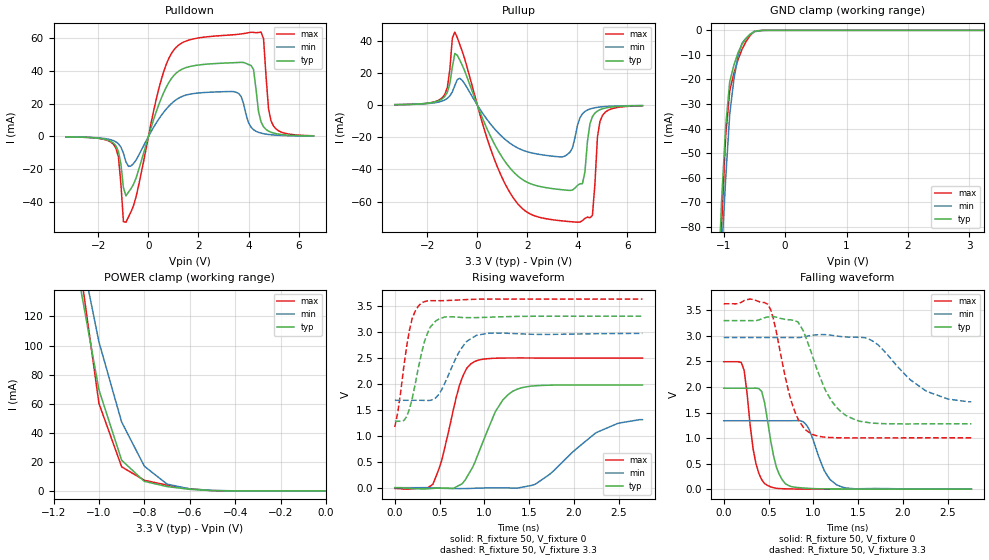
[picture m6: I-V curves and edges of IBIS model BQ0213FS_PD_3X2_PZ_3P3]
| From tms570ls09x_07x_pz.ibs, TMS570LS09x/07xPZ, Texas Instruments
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|   Model Cell BQ0213FS_PD_3X2_PZ_3P3
|BQ0213FS_PD_3X2_PZ_3P3
[Model]   BQ0213FS_PD_3X2_PZ_3P3
Model_type   I/O
Polarity   Non-Inverting
Enable   Active-Low
Vinl =  1.25
Vinh =  1.65
Cref =  15.0001pF
Rref =  101.0000M
Vref =  0V
Vmeas =  1.65
C_comp   1.2p   1.2p   1.2p
[Model Spec]
Vinl   1.25   1.12   1.38
Vinh   1.65   1.45   1.75
[Temperature Range]   25   155   -40
[Voltage Range]   3.3   2.97   3.63
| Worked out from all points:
|   slope of the pulldown table from 0 to 0.495 V, typ, clamps not added: 22 ohm
|   slope of the pullup table from 0 to 0.495 V, typ, clamps not added: 26.9 ohm
|   GND clamp passes 1 mA (typ) near -0.53 V on its own axis
|   POWER clamp passes 1 mA (typ) near -0.59 V on its own axis
|   rising waveform, R_fixture 50, V_fixture 0: 20-80 % time 297ps typ, 507ps min, 210ps max; typ from 0 V to 1.98 V
|   rising waveform, R_fixture 50, V_fixture 3.3: 20-80 % time 159ps typ, 218ps min, 127ps max; typ from 1.28 V to 3.3 V
|   falling waveform, R_fixture 50, V_fixture 0: 20-80 % time 129ps typ, 181ps min, 108ps max; typ from 1.98 V to 0.001 V
|   falling waveform, R_fixture 50, V_fixture 3.3: 20-80 % time 290ps typ, 442ps min, 208ps max; typ from 3.3 V to 1.28 V
[POWER_clamp]
|   voltage   I(typ)   I(min)   I(max)
-3.3V     2.375A     2.63A      3.153A
-1.1V     156mA      180.2mA    173.4mA
-1.067V   127.2mA    154.3mA    135.6mA
-1.033V   98.41mA    128.4mA    97.92mA
-1V       69.61mA    102.5mA    60.2mA
-900mV    21.13mA    47.41mA    16.61mA
-800mV    6.576mA    17mA       7.309mA
-700mV    2.999mA    4.688mA    3.99mA
-600mV    1.087mA    1.404mA    1.425mA
-500mV    187uA      358.1uA    203.4uA
0V        311.4pA    5.945nA    272.3pA
[Pulldown]
|   voltage   I(typ)   I(min)   I(max)
-3.3V     -269.8uA   -248.1uA   -260.2uA
-1.4V     -4.056mA   -2.548mA   -4.78mA
-1.2V     -9.104mA   -4.482mA   -12.53mA
-900mV    -36.12mA   -15.43mA   -52.08mA
1V        36.78mA    21.07mA    52.28mA
3.5V      44.86mA    26.92mA    61.93mA
4.1V      43.14mA    5.644mA    63.29mA
4.5V      8.805mA    2.025mA    63.4mA
4.6V      5.861mA    1.678mA    59.29mA
4.8V      3.241mA    1.203mA    16.69mA
5V        2.072mA    900.6uA    6.272mA
6.6V      302.2uA    232.4uA    414.2uA
[Pullup]
|   voltage   I(typ)   I(min)   I(max)
-3.3V     296.7uA    284.3uA    270.4uA
-1.4V     3.996mA    2.582mA    4.655mA
-1.2V     8.017mA    4.201mA    10.97mA
-900mV    32.15mA    12.24mA    45.44mA
1.4V      -40.82mA   -24.72mA   -56.86mA
3.4V      -52.65mA   -32.22mA   -72.03mA
4V        -49.98mA   -12.64mA   -72.82mA
4.2V      -48.91mA   -5.386mA   -71.83mA
4.6V      -7.16mA    -1.965mA   -68.52mA
4.8V      -3.684mA   -1.373mA   -19.8mA
5V        -2.282mA   -1.01mA    -6.487mA
6.6V      -316.6uA   -254.8uA   -401.1uA
[GND_clamp]
|   voltage   I(typ)   I(min)   I(max)
-3.3V     -1.947A    -1.623A    -3.254A
-1.1V     -112mA     -127mA     -135.8mA
-1.033V   -69.61mA   -91.63mA   -80.19mA
-966.7mV  -39.23mA   -60.62mA   -43.11mA
-900mV    -20.86mA   -34.02mA   -24.52mA
-833.3mV  -14.26mA   -20.12mA   -17.61mA
-766.7mV  -9.194mA   -10.52mA   -12.01mA
-700mV    -5.668mA   -5.208mA   -7.706mA
-566.7mV  -1.566mA   -1.573mA   -2.055mA
-500mV    -402.3uA   -585.8uA   -459.7uA
-300mV    -821.9nA   -7.17uA    -404.6nA
3.233V    296.5pA    4.008uA    206.9pA
[Ramp]
| variable   typ   min   max
dV/dt_f   1.26115/0.2950033n  0.8126168/0.4782827n   1.631567/0.2134149n
dV/dt_r   1.201273/0.3013661n  0.8158071/0.535569n   1.515362/0.2079949n
R_load = 50
[Rising Waveform]
R_fixture = 50
V_fixture = 0
V_fixture_min = 0
V_fixture_max = 0
|   time   V(typ)   V(min)   V(max)
0s        -29.41uV   10.5uV     -14.61mV
424ps     -14.21mV   -3.24mV    63.63mV
524ps     -7.849mV   -11.94mV   525.3mV
720ps     47.03mV    -17.96mV   1.958V
888ps     465mV      -11.29mV   2.425V
1.124ns   1.469V     -3.041mV   2.491V
1.312ns   1.852V     -6.722mV   2.496V
1.568ns   1.961V     66.56mV    2.496V
2.24ns    1.977V     1.051V     2.495V
2.764ns   1.977V     1.309V     2.495V
[Rising Waveform]
R_fixture = 50
V_fixture = 3.3
V_fixture_min = 2.97
V_fixture_max = 3.63
|   time   V(typ)   V(min)   V(max)
0s        1.281V     1.682V     1.167V
100ps     1.291V     1.682V     2.323V
164ps     1.514V     1.682V     3.034V
228ps     1.997V     1.682V     3.398V
296ps     2.569V     1.681V     3.557V
392ps     3.082V     1.679V     3.599V
456ps     3.207V     1.728V     3.599V
720ps     3.279V     2.619V     3.613V
912ps     3.274V     2.933V     3.627V
2.764ns   3.3V       2.969V     3.63V
[Falling Waveform]
R_fixture = 50
V_fixture = 0
V_fixture_min = 0
V_fixture_max = 0
|   time   V(typ)   V(min)   V(max)
0s        1.977V     1.34V      2.495V
228ps     1.977V     1.34V      2.328V
360ps     1.978V     1.34V      500.7mV
492ps     1.314V     1.34V      70.79mV
588ps     431.1mV    1.34V      17.06mV
752ps     51.38mV    1.34V      4.516mV
912ps     19.49mV    1.28V      1.155mV
1.124ns   5.67mV     357.7mV    629.4uV
1.312ns   2.257mV    48.54mV    831.6uV
2.764ns   537.6uV    541.3uV    34.65uV
[Falling Waveform]
R_fixture = 50
V_fixture = 3.3
V_fixture_min = 2.97
V_fixture_max = 3.63
|   time   V(typ)   V(min)   V(max)
0s        3.3V       2.97V      3.63V
492ps     3.371V     2.97V      3.621V
752ps     3.316V     2.97V      1.732V
828ps     3.276V     2.969V     1.378V
976ps     2.684V     3.01V      1.082V
1.208ns   1.716V     3.012V     1.01V
1.464ns   1.362V     2.976V     1.004V
1.724ns   1.287V     2.825V     1.005V
2.264ns   1.279V     1.916V     1.006V
2.764ns   1.28V      1.711V     1.006V
